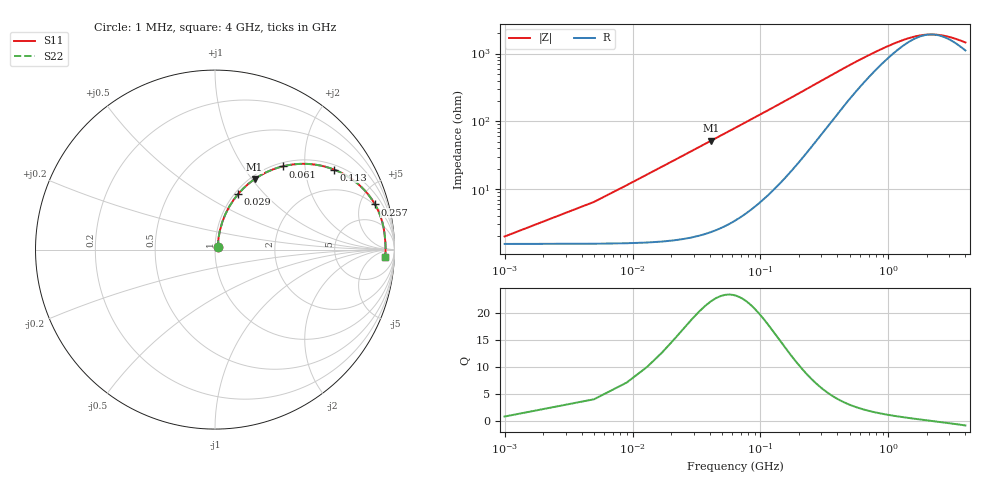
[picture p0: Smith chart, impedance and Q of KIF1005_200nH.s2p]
!version-2
!date-12.2020
!Series
# MHz S RI R 50
!Freq ReS11 ImS11 ReS21 ImS21 ReS12 ImS12 ReS22 ImS22
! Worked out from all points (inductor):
!   1001 points, 1 MHz to 4 GHz, reference 50 ohm
!   read as one part in series: L = 200 nH near 21 MHz
!   highest Q = 21.9 at 41 MHz (marker M1), where L = 200 nH
!   self-resonance near 2.166 GHz
!   S11 on the Smith chart (normalised r, x): 1 MHz: 1.03, +0.03; 29 MHz: 1.04, +0.73; 61 MHz: 1.07, +1.53; 113 MHz: 1.16, +2.87; 257 MHz: 1.89, +6.70; 4 GHz: 23, -19
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1  0.0154 0.0122  0.9846 -0.0122  0.9846 -0.0122  0.0154 0.0122
13  0.0407 0.1539  0.9593 -0.1539  0.9593 -0.1539  0.0407 0.1539
25  0.103 0.2762  0.897 -0.2762  0.897 -0.2762  0.103 0.2762
29  0.1298 0.3106  0.8702 -0.3106  0.8702 -0.3106  0.1298 0.3106
41  0.2201 0.3924  0.7799 -0.3924  0.7799 -0.3924  0.2201 0.3924
49  0.2836 0.4297  0.7164 -0.4297  0.7164 -0.4297  0.2836 0.4297
61  0.3762 0.4636  0.6238 -0.4636  0.6238 -0.4636  0.3762 0.4636
85  0.534 0.4761  0.466 -0.4761  0.466 -0.4761  0.534 0.4761
113  0.6646 0.4453  0.3354 -0.4453  0.3354 -0.4453  0.6646 0.4453
141  0.7503 0.4009  0.2497 -0.4009  0.2497 -0.4009  0.7503 0.4009
173  0.8131 0.3511  0.1869 -0.3511  0.1869 -0.3511  0.8131 0.3511
257  0.8914 0.2518  0.1086 -0.2518  0.1086 -0.2518  0.8914 0.2518
341  0.9203 0.1901  0.0797 -0.1901  0.0797 -0.1901  0.9203 0.1901
437  0.934 0.1456  0.066 -0.1456  0.066 -0.1456  0.934 0.1456
669  0.9445 0.0889  0.0555 -0.0889  0.0555 -0.0889  0.9445 0.0889
973  0.948 0.0539  0.052 -0.0539  0.052 -0.0539  0.948 0.0539
1337  0.9496 0.0305  0.0504 -0.0305  0.0504 -0.0305  0.9496 0.0305
1653  0.9501 0.0167  0.0499 -0.0167  0.0499 -0.0167  0.9501 0.0167
2001  0.9503 0.00484  0.0497 -0.00484  0.0497 -0.00484  0.9503 0.00484
2669  0.9502 -0.0129  0.0498 0.0129  0.0498 0.0129  0.9502 -0.0129
3337  0.9496 -0.0273  0.0504 0.0273  0.0504 0.0273  0.9496 -0.0273
4000  0.9487 -0.04  0.0513 0.04  0.0513 0.04  0.9487 -0.04
